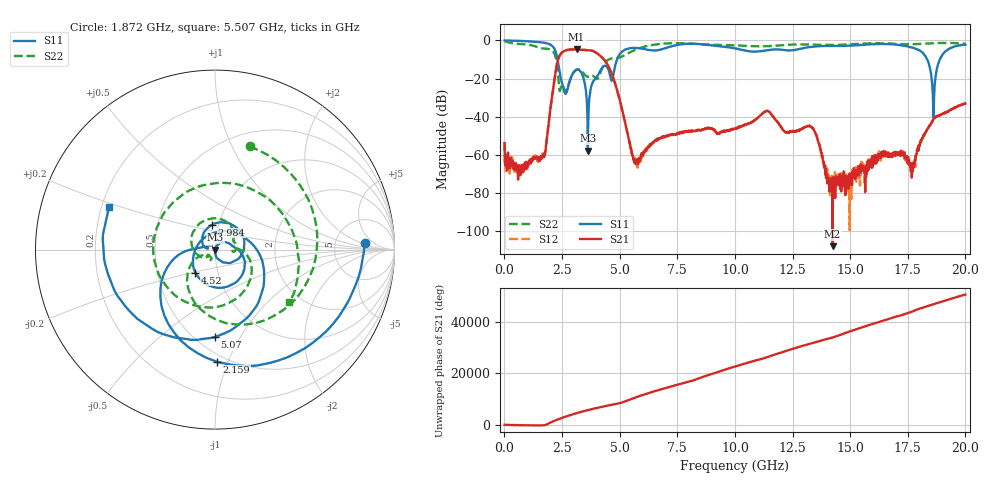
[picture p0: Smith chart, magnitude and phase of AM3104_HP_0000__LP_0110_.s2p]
!Created with skrf (http://scikit-rf.org).
# Hz S RI R 50.0
!freq ReS11 ImS11 ReS21 ImS21 ReS12 ImS12 ReS22 ImS22
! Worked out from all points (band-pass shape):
!   1601 points, 10 MHz to 20 GHz, reference 50 ohm
!   highest |S21| = -4.68 dB at 3.133 GHz (marker M1); lowest = -107.9 dB at 14.24 GHz (marker M2)
!   |S21| within 3 dB of the highest: 2.408 GHz to 4.121 GHz (1.713 GHz wide, 52.5 % of centre)
!   lowest |S11| = -57.8 dB at 3.621 GHz (marker M3), VSWR 1.00, Z = 50.1 - j0.0873 ohm
!   |S11| at or under -10 dB: 2.307 GHz to 4.888 GHz (2.581 GHz wide, 71.7 % of centre); 18.34 GHz to 18.89 GHz (540.5 MHz wide, 2.9 % of centre)
!   |S22| runs from -26.8 to -0.2 dB; largest |S21 - S12| = 0.0049
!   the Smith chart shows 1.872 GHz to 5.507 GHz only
!   S11 on the Smith chart (normalised r, x): 1.872 GHz: 10, +3; 2.159 GHz: 0.45, -0.91; 2.984 GHz: 0.93, +0.26; 4.52 GHz: 0.78, -0.21; 5.07 GHz: 0.62, -0.79; 5.507 GHz: 0.23, +0.19
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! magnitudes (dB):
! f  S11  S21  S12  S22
! 10 MHz  0.0  -53.9  -53.4  -0.2
! 684.7 MHz  -0.2  -69.7  -66.1  -1.8
! 1.672 GHz  -1.1  -61.2  -60.3  -4.2
! 1.872 GHz  -1.6  -48.6  -48.6  -4.3
! 2.159 GHz  -4.1  -21.5  -21.5  -6.6
! 2.621 GHz  -27.4  -5.4  -5.4  -26.1
! 2.984 GHz  -17.1  -4.7  -4.7  -17.1
! 3.133 GHz  -15.4  -4.7  -4.7  -15.4
! 3.346 GHz  -16.9  -4.9  -4.9  -16.0
! 3.621 GHz  -57.8  -5.1  -5.1  -18.9
! 4.52 GHz  -15.5  -13.7  -13.6  -9.9
! 5.07 GHz  -6.2  -34.4  -34.3  -8.6
! 5.507 GHz  -3.9  -56.9  -57.8  -5.9
! 6.682 GHz  -5.0  -52.0  -51.8  -1.9
! 10.01 GHz  -4.1  -46.0  -46.3  -2.5
! 13.34 GHz  -3.3  -45.6  -45.5  -2.2
! 14.24 GHz  -2.9  -107.9  -77.3  -2.3
! 16.68 GHz  -1.9  -59.3  -58.8  -1.6
! 17.7 GHz  -3.8  -64.2  -66.5  -1.9
! 18.61 GHz  -40.8  -41.4  -41.4  -1.4
! 19.03 GHz  -7.1  -38.2  -38.4  -1.2
! 20 GHz  -2.2  -33.1  -33.0  -1.7
